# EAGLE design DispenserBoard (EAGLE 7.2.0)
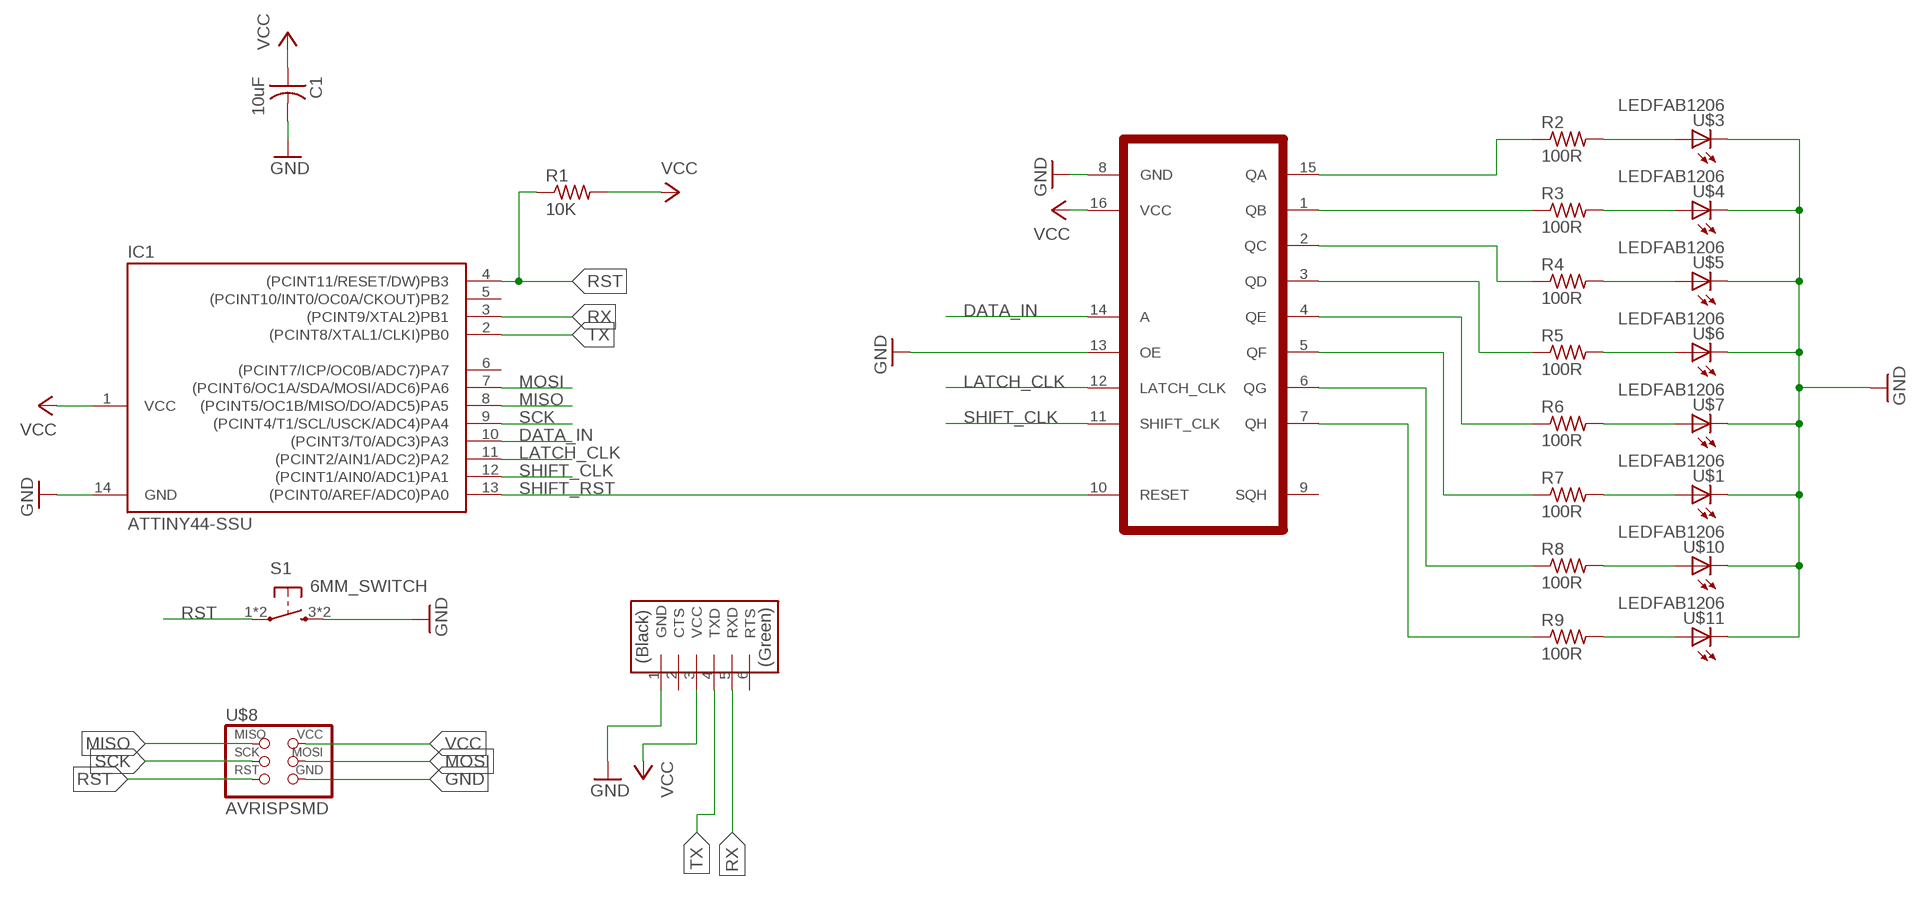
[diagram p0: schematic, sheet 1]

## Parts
C1  10uF  CAP-US1206FAB  [C1206FAB]
IC1  ATTINY44-SSU  [SOIC14]
R1  10K  RES-US1206FAB  [R1206FAB]
R2  100R  RES-US1206FAB  [R1206FAB]
R3  100R  RES-US1206FAB  [R1206FAB]
R4  100R  RES-US1206FAB  [R1206FAB]
R5  100R  RES-US1206FAB  [R1206FAB]
R6  100R  RES-US1206FAB  [R1206FAB]
R7  100R  RES-US1206FAB  [R1206FAB]
R8  100R  RES-US1206FAB  [R1206FAB]
R9  100R  RES-US1206FAB  [R1206FAB]
S1  6MM_SWITCH  [6MM_SWITCH]
U$1  LEDFAB1206  [LED1206FAB]
U$2  74HC595MC74HC595ADG  [SOIC16]
U$3  LEDFAB1206  [LED1206FAB]
U$4  LEDFAB1206  [LED1206FAB]
U$5  LEDFAB1206  [LED1206FAB]
U$6  LEDFAB1206  [LED1206FAB]
U$7  LEDFAB1206  [LED1206FAB]
U$8  AVRISPSMD  [2X03SMD]
U$9  FTDI-SMD-HEADER  [1X06SMD]
U$10  LEDFAB1206  [LED1206FAB]
U$11  LEDFAB1206  [LED1206FAB]

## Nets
DATA_IN: IC1.10((PCINT3/T0/ADC3)PA3) U$2.14(A)
GND: C1.2 IC1.14(GND) S1.3(S) S1.4(S) U$1.2(C) U$2.8(GND) U$2.13(OE) U$3.2(C) U$4.2(C) U$5.2(C) U$6.2(C) U$7.2(C) U$8.6(GND) U$9.1(GND) U$10.2(C) U$11.2(C)
LATCH_CLK: IC1.11((PCINT2/AIN1/ADC2)PA2) U$2.12(LATCH_CLK)
MISO: IC1.8((PCINT5/OC1B/MISO/DO/ADC5)PA5) U$8.1(MISO)
MOSI: IC1.7((PCINT6/OC1A/SDA/MOSI/ADC6)PA6) U$8.4(MOSI)
N$3: R7.2 U$1.1(A)
N$4: R8.2 U$10.1(A)
N$5: R9.2 U$11.1(A)
N$6: R2.1 U$2.15(QA)
N$7: R3.1 U$2.1(QB)
N$8: R2.2 U$3.1(A)
N$9: R3.2 U$4.1(A)
N$10: R4.2 U$5.1(A)
N$11: R5.2 U$6.1(A)
N$12: R6.2 U$7.1(A)
N$13: R4.1 U$2.2(QC)
N$14: R5.1 U$2.3(QD)
N$15: R6.1 U$2.4(QE)
N$16: R7.1 U$2.5(QF)
N$17: R8.1 U$2.6(QG)
N$18: R9.1 U$2.7(QH)
RST: IC1.4((PCINT11/RESET/DW)PB3) R1.1 S1.1(P) S1.2(P) U$8.5(RST)
RX: IC1.3((PCINT9/XTAL2)PB1) U$9.5(RXD)
SCK: IC1.9((PCINT4/T1/SCL/USCK/ADC4)PA4) U$8.3(SCK)
SHIFT_CLK: IC1.12((PCINT1/AIN0/ADC1)PA1) U$2.11(SHIFT_CLK)
SHIFT_RST: IC1.13((PCINT0/AREF/ADC0)PA0) U$2.10(RESET)
TX: IC1.2((PCINT8/XTAL1/CLKI)PB0) U$9.4(TXD)
VCC: C1.1 IC1.1(VCC) R1.2 U$2.16(VCC) U$8.2(VCC) U$9.3(VCC)
Unconnected: IC1.5((PCINT10/INT0/OC0A/CKOUT)PB2) IC1.6((PCINT7/ICP/OC0B/ADC7)PA7) U$2.9(SQH) U$9.2(CTS) U$9.6(RTS)

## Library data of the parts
C1 = fab:CAP-US
IC1 = fab:ATTINY44
R1-R9 = fab:RES-US: Resistor (US Symbol)
S1 = fab:6MM_SWITCH: OMRON SWITCH
U$1 U$3-U$7 U$10 U$11 = fab:LED: LED
U$2 = challenger:74HC595
U$8 = fab:AVRISP
U$9 = fab:FTDI-SMD-HEADER

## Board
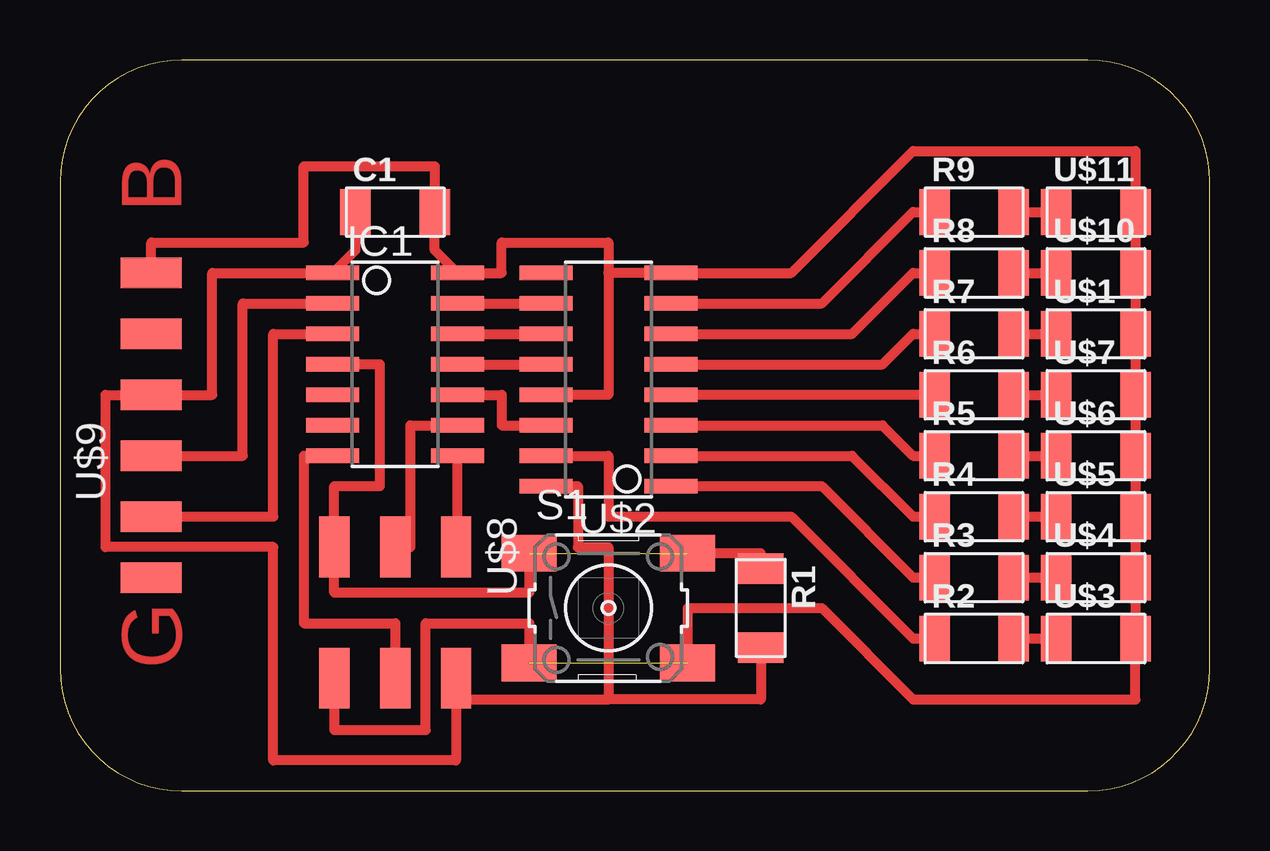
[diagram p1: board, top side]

Size 47.93 x 30.47 mm. Coordinates in mm from the lower left corner, seen from the top.
Outline: 47.93,5.08 47.93,25.39 arc90 42.85,30.47 5.08,30.47 arc90 0,25.39 0,5.08 arc90 5.08,0 42.85,0 arc90 47.93,5.08
Copper layers (1*16): Top 0.035mm / dielectric 1.5mm / Bottom 0.035mm
Design rules "fabmodule": minimum track width 10mil, minimum drill 0.4mm, track to track 0.42mm, track to pad 0.42mm, pad to pad 0.42mm, via to via 0.42mm, smd to smd 0.42mm, copper to edge 40mil, drill to drill 0.8mm, minimum pad ring 10mil, minimum via ring 8mil, stop-mask expansion 4mil, vias tented up to drill 0mil, thermal gap 10mil

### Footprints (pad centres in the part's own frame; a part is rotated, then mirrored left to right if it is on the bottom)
C1206FAB = smd 1.27 x 1.905: 1 -1.651,0; 2 1.651,0
SOIC14 = smd 0.61 x 2.21: 1 -3.81,-2.603; 2 -2.54,-2.603; 3 -1.27,-2.603; 4 0,-2.603; 5 1.27,-2.603; 6 2.54,-2.603; 7 3.81,-2.603; 8 3.81,2.603; 9 2.54,2.603; 10 1.27,2.603; 11 0,2.603; 12 -1.27,2.603; 13 -2.54,2.603; 14 -3.81,2.603
R1206FAB = smd 1.27 x 1.905: 1 -1.651,0; 2 1.651,0
6MM_SWITCH = smd 2.286 x 1.524: 1 -3.302,2.286; 2 3.302,2.286; 3 -3.302,-2.286; 4 3.302,-2.286
LED1206FAB = smd 1.27 x 1.905: 1 -1.651,0; 2 1.651,0
SOIC16 = smd 0.61 x 2.21: 1 -3.81,-2.603; 2 -2.54,-2.603; 3 -1.27,-2.603; 4 0,-2.603; 5 1.27,-2.603; 6 2.54,-2.603; 7 3.81,-2.603; 8 5.08,-2.603; 9 5.08,2.603; 10 3.81,2.603; 11 2.54,2.603; 12 1.27,2.603; 13 0,2.603; 14 -1.27,2.603; 15 -2.54,2.603; 16 -3.81,2.603
2X03SMD = smd 2.54 x 1.27: 1 -2.54,2.54; 2 2.92,2.54; 3 -2.54,0; 4 2.92,0; 5 -2.54,-2.54; 6 2.92,-2.54
1X06SMD = smd 2.54 x 1.27: 1 0,6.35; 2 0,3.81; 3 0,1.27; 4 0,-1.27; 5 0,-3.81; 6 0,-6.35

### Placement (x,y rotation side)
C1  13.97,24.13 0 top
IC1  13.97,17.78 270 top
R1  29.21,7.62 270 top
R2  38.1,6.35 0 top
R3  38.1,8.89 0 top
R4  38.1,11.43 0 top
R5  38.1,13.97 0 top
R6  38.1,16.51 0 top
R7  38.1,19.05 0 top
R8  38.1,21.59 0 top
R9  38.1,24.13 0 top
S1  22.86,7.62 0 top
U$1  43.18,19.05 0 top
U$2  22.86,16.51 90 top
U$3  43.18,6.35 0 top
U$4  43.18,8.89 0 top
U$5  43.18,11.43 0 top
U$6  43.18,13.97 0 top
U$7  43.18,16.51 0 top
U$8  13.97,7.62 270 top
U$9  3.81,15.24 0 top
U$10  43.18,21.59 0 top
U$11  43.18,24.13 0 top

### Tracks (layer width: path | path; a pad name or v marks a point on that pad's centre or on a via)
DATA_IN
  Top 0.406: IC1.10 18.41,16.51 18.41,15.24 U$2.14
GND  (1 unrouted)
  Top 0.406: U$8.6 11.43,2.54 15.24,2.54 15.24,6.99 19.56,6.99 S1.3 | 22.86,21.59 22.86,16.51 U$2.13 | U$2.8 22.86,21.59 | U$2.8 25.4,21.59 | 22.86,21.59 22.86,22.86 18.41,22.86 18.41,21.59 IC1.14 15.62,22.54 C1.2 15.62,26.04 10.16,26.04 10.16,22.86 3.81,22.86 U$9.1 | U$2.8 30.48,21.59 35.56,26.67 44.83,26.67 U$11.2 U$10.2 U$1.2 U$7.2 U$6.2 U$5.2 U$4.2 U$3.2 44.83,3.81 35.56,3.81 31.75,7.62 26.16,7.62 S1.4
LATCH_CLK
  Top 0.406: IC1.11 U$2.12
MISO
  Top 0.406: U$8.1 16.57,10.16 IC1.8
MOSI
  Top 0.406: IC1.7 10.16,13.97 10.16,6.99 13.97,6.99 U$8.4
N$3
  Top 0.406: R7.2 U$1.1
N$4
  Top 0.406: R8.2 U$10.1
N$5
  Top 0.406: R9.2 U$11.1
N$6
  Top 0.406: U$2.15 22.86,13.97 22.86,11.43 30.48,11.43 35.56,6.35 R2.1
N$7
  Top 0.406: U$2.1 31.75,12.7 35.56,8.89 R3.1
N$8
  Top 0.406: R2.2 U$3.1
N$9
  Top 0.406: R3.2 U$4.1
N$10
  Top 0.406: R4.2 U$5.1
N$11
  Top 0.406: R5.2 U$6.1
N$12
  Top 0.406: R6.2 U$7.1
N$13
  Top 0.406: U$2.2 33.02,13.97 35.56,11.43 R4.1
N$14
  Top 0.406: U$2.3 34.29,15.24 35.56,13.97 R5.1
N$15
  Top 0.406: R6.1 U$2.4
N$16
  Top 0.406: U$2.5 34.29,17.78 35.56,19.05 R7.1
N$17
  Top 0.406: U$2.6 33.02,19.05 35.56,21.59 R8.1
N$18
  Top 0.406: U$2.7 31.75,20.32 35.56,24.13 R9.1
RST  (1 unrouted)
  Top 0.406: IC1.4 13.34,17.78 13.34,12.7 11.43,12.7 U$8.5 11.43,8.26 19.56,8.26 S1.1 | R1.1 29.21,9.91 S1.2
RX
  Top 0.406: U$9.5 8.89,11.43 8.89,19.05 IC1.3
SCK
  Top 0.406: U$8.3 14.61,10.16 14.61,15.24 IC1.9
SHIFT_CLK
  Top 0.406: IC1.12 U$2.11
SHIFT_RST
  Top 0.406: IC1.13 U$2.10
TX
  Top 0.406: U$9.4 7.62,13.97 7.62,20.32 IC1.2
VCC
  Top 0.406: R1.2 29.21,3.81 22.86,3.81 | U$2.16 21.59,12.7 21.59,10.16 22.86,10.16 22.86,3.81 | 22.86,3.81 16.51,3.81 U$8.2 16.51,1.27 8.89,1.27 8.89,10.16 1.91,10.16 1.91,16.51 U$9.3 6.35,16.51 6.35,21.59 IC1.1 12.32,22.54 C1.1

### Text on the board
Top: B | G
